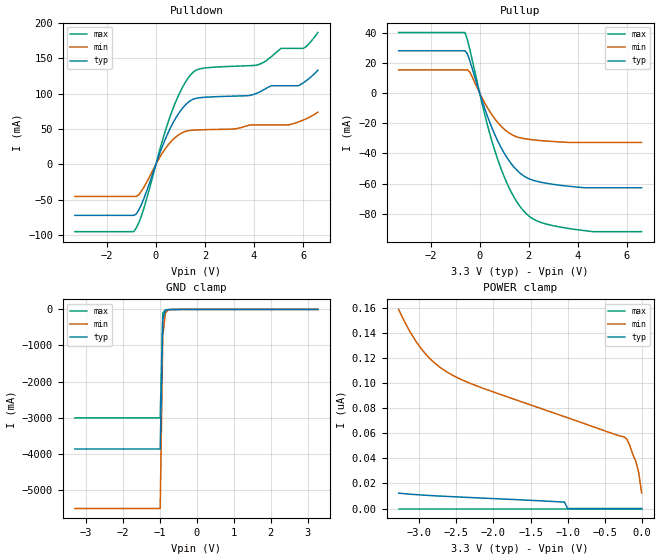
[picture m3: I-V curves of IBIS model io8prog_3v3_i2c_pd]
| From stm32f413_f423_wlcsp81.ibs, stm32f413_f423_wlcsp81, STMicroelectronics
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[Model]  io8prog_3v3_i2c_pd
Model_type I/O
Polarity   Non-Inverting
Enable   Active-Low
Vinl =   0.540000V
Vinh =   1.260000V
Vmeas =  0.900000V
Cref =   100.000000pF
Rref =   1.000000k
Vref =   1.800000V
C_comp   2.577900pF   2.407400pF   2.792100pF
[Temperature Range]   25.000000   0.125000k   -40.000000
[Pullup Reference]   3.300000V   2.700000V   3.600000V
[Pulldown Reference]   0.0V   0.0V   0.0V
[POWER Clamp Reference]   3.300000V   2.700000V   3.600000V
[GND Clamp Reference]   0.0V   0.0V   0.0V
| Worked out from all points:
|   slope of the pulldown table from 0 to 0.495 V, typ, clamps not added: 11.1 ohm
|   slope of the pullup table from 0 to 0.495 V, typ, clamps not added: 21.7 ohm
|   GND clamp passes 1 mA (typ) near -0.57 V on its own axis
[Pulldown]
|Voltage   I(typ)   I(min)   I(max)
-3.3V     -72.2mA    -45.43mA   -95.28mA
-900mV    -72.2mA    -45.43mA   -95.28mA
-500mV    -49.3mA    -32.97mA   -63.37mA
200mV     19.69mA    12.49mA    25.95mA
600mV     52.23mA    31.69mA    69.99mA
1.1V      80.2mA     45.29mA    110.3mA
1.5V      91.99mA    48.41mA    130mA
4.2V      102.1mA    55.95mA    141.6mA
5.1V      111.4mA    55.95mA    164.3mA
5.8V      111.4mA    59.96mA    164.3mA
6.1V      117.8mA    64.19mA    166.1mA
6.6V      133.3mA    73.83mA    186.7mA
[Pullup]
|Voltage   I(typ)   I(min)   I(max)
-3.3V     27.94mA    15.3mA     39.98mA
-600mV    27.94mA    15.3mA     39.98mA
-500mV    25.89mA    15.3mA     35.29mA
-400mV    21.3mA     13.82mA    28.75mA
300mV     -14.62mA   -9.248mA   -20.15mA
800mV     -33.8mA    -20.67mA   -46.89mA
1.1V      -42.41mA   -25.27mA   -59.19mA
1.4V      -49.01mA   -28.29mA   -68.91mA
2V        -56.64mA   -30.64mA   -81.32mA
2.6V      -59.37mA   -31.63mA   -86.15mA
3.9V      -62.11mA   -32.7mA    -90.24mA
6.6V      -62.7mA    -32.7mA    -91.7mA
[GND_clamp]
|Voltage   I(typ)   I(min)   I(max)
-3.3V     -3.872A    -5.523A    -3.009A
-990mV    -3.872A    -5.523A    -3.009A
-920mV    -262.2mA   -719.6mA   -104.3mA
-850mV    -25.2mA    -101mA     -13.09mA
-780mV    -6.971mA   -18.01mA   -7.205mA
3.28V     81.28uA    57.88uA    93.99uA
[POWER_clamp]
|Voltage   I(typ)   I(min)   I(max)
-3.28V    12.28nA    159nA      0A
-3.12V    11.42nA    140.5nA    0A
-2.96V    10.74nA    126.5nA    0A
-2.76V    10.06nA    114.5nA    0A
-2.56V    9.465nA    106.7nA    0A
-1.04V    5.098nA    73.34nA    0A
-1V       0A         72.52nA    0A
-240mV    0A         57.28nA    0A
-200mV    0A         55.46nA    0A
-80mV     0A         38nA       0A
-40mV     0A         29.01nA    0A
0V        0A         12.48nA    0A
[Ramp]
| variable   typ   min   max
dV/dt_r  1.29804/6.00000u   0.82818/6.00000u   1.59294/6.00000u
dV/dt_f  1.60754/6.00000u   1.14540/6.00000u   1.84948/6.00000u
R_load = 50.000000
